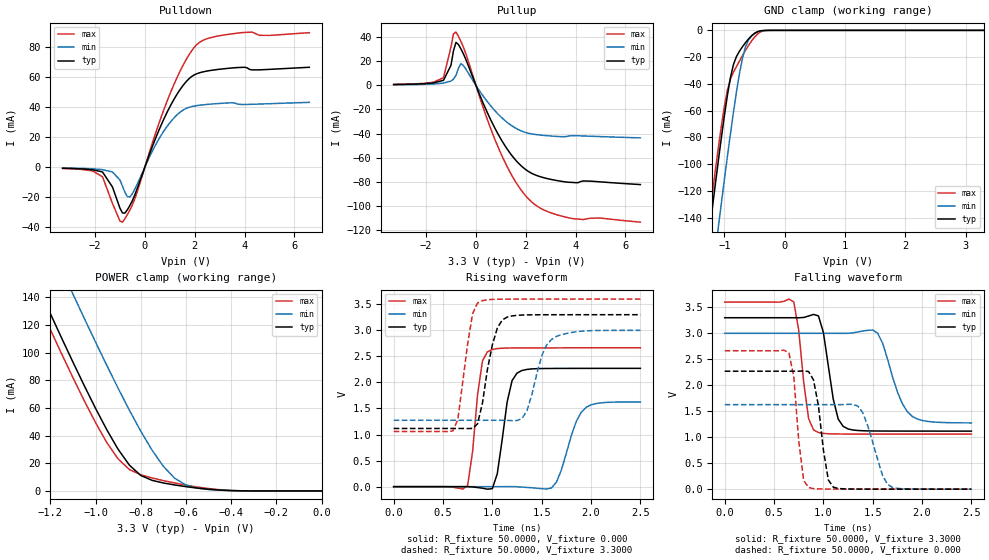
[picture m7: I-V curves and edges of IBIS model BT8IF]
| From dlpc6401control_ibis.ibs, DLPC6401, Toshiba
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[Model]   BT8IF
Model_type   3-state
Polarity   Non-Inverting
Enable   Active-Low
C_comp   1.404pF   NA   NA
Vmeas = 1.40V
|Variable   typ   min   max
[Voltage range]  3.3   3.0   3.6
[Temperature Range]   25.0000   125.000   0.000
[Pullup Reference]   3.3000V   3.0000V   3.6000V
[Pulldown Reference]   0.000V   0.000V   0.000V
[POWER Clamp Reference]   3.3000V   3.0000V   3.6000V
[GND Clamp Reference]   0.000V   0.000V   0.000V
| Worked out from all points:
|   slope of the pulldown table from 0 to 0.495 V, typ, clamps not added: 22.7 ohm
|   slope of the pullup table from 0 to 0.495 V, typ, clamps not added: 20.5 ohm
|   GND clamp passes 1 mA (typ) near -0.45 V on its own axis
|   POWER clamp passes 1 mA (typ) near -0.48 V on its own axis
|   rising waveform, R_fixture 50.0000, V_fixture 0.000: 20-80 % time 108ps typ, 164ps min, 89.5ps max; typ from 0 V to 2.27 V
|   rising waveform, R_fixture 50.0000, V_fixture 3.3000: 20-80 % time 129ps typ, 158ps min, 111ps max; typ from 1.12 V to 3.3 V
|   falling waveform, R_fixture 50.0000, V_fixture 3.3000: 20-80 % time 111ps typ, 183ps min, 88.2ps max; typ from 3.3 V to 1.12 V
|   falling waveform, R_fixture 50.0000, V_fixture 0.000: 20-80 % time 97.4ps typ, 157ps min, 74.7ps max; typ from 2.27 V to 0 V
[Pulldown]
| voltage   I(typ)   I(min)   I(max)
-3.3V     -738.7uA   -567.3uA   -926.4uA
-2.1V     -1.741mA   -1.126mA   -2.525mA
-1.7V     -3.22mA    -1.677mA   -6.426mA
-1.3V     -13.22mA   -3.242mA   -24.14mA
-900mV    -30.46mA   -12.55mA   -36.67mA
-600mV    -25.54mA   -19.84mA   -28.53mA
400mV     17.91mA    13.84mA    21.06mA
950mV     38.44mA    28.43mA    46.36mA
1.55V     54.75mA    38.17mA    68.36mA
2.05V     61.95mA    40.87mA    81.01mA
3.8V      66.37mA    41.82mA    89.39mA
6.6V      66.5mA     43.14mA    89.56mA
[Pullup]
| voltage   I(typ)   I(min)   I(max)
-3.3V     610.1uA    402.9uA    732.5uA
-1.3V     4.103mA    1.768mA    6.279mA
-1V       16.51mA    3.497mA    31.64mA
-900mV    28.48mA    5.029mA    42.54mA
-800mV    35.48mA    8.195mA    44mA
-600mV    30.1mA     17.92mA    36.22mA
-500mV    25.95mA    16.3mA     31.45mA
950mV     -42.6mA    -25.09mA   -53.98mA
1.55V     -60.85mA   -34.96mA   -78.43mA
2.1V      -71.2mA    -39.67mA   -93.79mA
3.7V      -80.23mA   -42.08mA   -109.6mA
6.6V      -82.16mA   -43.54mA   -113.3mA
[GND_clamp]
| voltage   I(typ)   I(min)   I(max)
-3.3V     -944.9mA   -993.5mA   -933.7mA
-1.3V     -169.6mA   -220.5mA   -158.5mA
-1.25V    -151.2mA   -201.9mA   -140.2mA
-1.2V     -132.9mA   -183.4mA   -122.2mA
-1.1V     -97.21mA   -147mA     -87.47mA
-1V       -63.63mA   -111.4mA   -56.62mA
-900mV    -35.29mA   -77.26mA   -36.39mA
-800mV    -19.53mA   -45.93mA   -27.04mA
-700mV    -12.2mA    -20.73mA   -18.85mA
-600mV    -6.422mA   -7.153mA   -11.28mA
-450mV    -954.9uA   -1.183mA   -2.691mA
3.3V      2.119nA    24.26uA    12.22nA
[POWER_clamp]
| voltage   I(typ)   I(min)   I(max)
-3.3V     917.5mA    964.8mA    906.4mA
-1.3V     164.1mA    213.9mA    152.5mA
-1.25V    146mA      195.8mA    134.5mA
-1.2V     128.2mA    177.9mA    116.7mA
-1.1V     93.14mA    142.3mA    81.92mA
-950mV    44.15mA    90.68mA    34.95mA
-850mV    18.58mA    58.26mA    15.44mA
-750mV    7.652mA    29.46mA    9.374mA
-650mV    4.312mA    9.163mA    5.736mA
-600mV    3.088mA    4.252mA    4.184mA
-500mV    1.206mA    1.062mA    1.712mA
0V        2.118nA    56.3nA     15.39nA
[Ramp]
| variable   typ   min   max
dV/dt_r   1.3622/96.8321p   0.9756/0.1596n   1.5986/75.4260p
dV/dt_f   1.3096/0.1021n   1.0346/0.1784n   1.5245/78.0740p
R_load = 50.0000
[Rising Waveform]
R_fixture = 50.0000
V_fixture = 0.000
V_fixture_min = 0.000
V_fixture_max = 0.000
| time   V(typ)   V(min)   V(max)
0s        0V         0V         0V
750ps     187uV      1.409uV    24.75mV
900ps     -29.55mV   -6.973uV   2.413V
950ps     -48.14mV   -6.294uV   2.586V
1.05ns    247.9mV    30.92uV    2.65V
1.15ns    1.624V     393.3uV    2.66V
1.25ns    2.179V     -2.383mV   2.662V
1.6ns     2.268V     -24.61mV   2.664V
1.95ns    2.27V      1.521V     2.664V
2.5ns     2.27V      1.626V     2.664V
[Rising Waveform]
R_fixture = 50.0000
V_fixture = 3.3000
V_fixture_min = 3.0000
V_fixture_max = 3.6000
| time   V(typ)   V(min)   V(max)
0s        1.117V     1.274V     1.059V
600ps     1.117V     1.274V     1.071V
650ps     1.117V     1.274V     1.286V
800ps     1.118V     1.274V     3.321V
850ps     1.205V     1.274V     3.524V
1ns       2.72V      1.274V     3.593V
1.1ns     3.199V     1.273V     3.597V
1.35ns    3.296V     1.452V     3.599V
1.6ns     3.299V     2.825V     3.6V
2.5ns     3.3V       2.999V     3.6V
[Falling Waveform]
R_fixture = 50.0000
V_fixture = 3.3000
V_fixture_min = 3.0000
V_fixture_max = 3.6000
| time   V(typ)   V(min)   V(max)
0s        3.3V       3V         3.6V
700ps     3.3V       3V         3.604V
850ps     3.333V     3V         1.359V
950ps     3.336V     3V         1.09V
1.1ns     1.732V     3V         1.064V
1.2ns     1.209V     2.999V     1.062V
1.55ns    1.119V     3.002V     1.06V
1.75ns    1.118V     1.871V     1.06V
1.9ns     1.118V     1.401V     1.06V
2.5ns     1.117V     1.276V     1.059V
[Falling Waveform]
R_fixture = 50.0000
V_fixture = 0.000
V_fixture_min = 0.000
V_fixture_max = 0.000
| time   V(typ)   V(min)   V(max)
0s        2.271V     1.627V     2.664V
650ps     2.271V     1.627V     2.627V
700ps     2.27V      1.627V     2.173V
800ps     2.276V     1.627V     170.4mV
850ps     2.264V     1.627V     31.46mV
1.05ns    178.8mV    1.627V     2.796mV
1.1ns     39.49mV    1.627V     2.346mV
1.4ns     1.762mV    1.47V      992.1uV
1.7ns     844.4uV    34mV       419.4uV
2.5ns     150.5uV    473.4uV    72.06uV
